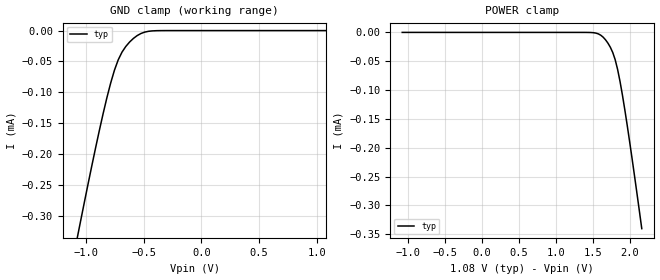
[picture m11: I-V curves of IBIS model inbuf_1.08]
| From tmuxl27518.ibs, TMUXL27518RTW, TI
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| inbuf_1.08
[Model]   inbuf_1.08
Model_type   Input
Vinl = 0.39
Vinh = 0.77
|   typ   min   max
C_comp   2.533030e-13   NA   NA
[Voltage Range]   1.08   NA   NA
[Temperature Range]   27   NA   NA
[Power Clamp Reference]   1.08   NA   NA
[GND Clamp Reference]   0   NA   NA
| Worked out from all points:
|   GND clamp passes 1 mA (typ) near -1.75 V on its own axis
[GND Clamp]
|   Voltage   I(typ)   I(min)   I(max)
-2.16V    -1.421mA   NA         NA
-1.08V    -340.4uA   NA         NA
-1.047V   -309.6uA   NA         NA
-883.6mV  -161.7uA   NA         NA
-818.2mV  -108.6uA   NA         NA
-752.7mV  -64.02uA   NA         NA
-720mV    -47.24uA   NA         NA
-654.5mV  -25.68uA   NA         NA
-589.1mV  -12.73uA   NA         NA
-523.6mV  -4.73uA    NA         NA
-360mV    -77.02nA   NA         NA
1.08V     74.72pA    NA         NA
[POWER Clamp]
|   Voltage   I(typ)   I(min)   I(max)
-1.08V    13.58nA    NA         NA
1.44V     -77.02nA   NA         NA
1.571V    -2.484uA   NA         NA
1.636V    -8.123uA   NA         NA
1.702V    -18.54uA   NA         NA
1.767V    -34.8uA    NA         NA
1.8V      -47.24uA   NA         NA
1.833V    -64.02uA   NA         NA
1.898V    -108.6uA   NA         NA
1.964V    -161.7uA   NA         NA
2.062V    -248.8uA   NA         NA
2.16V     -340.4uA   NA         NA
